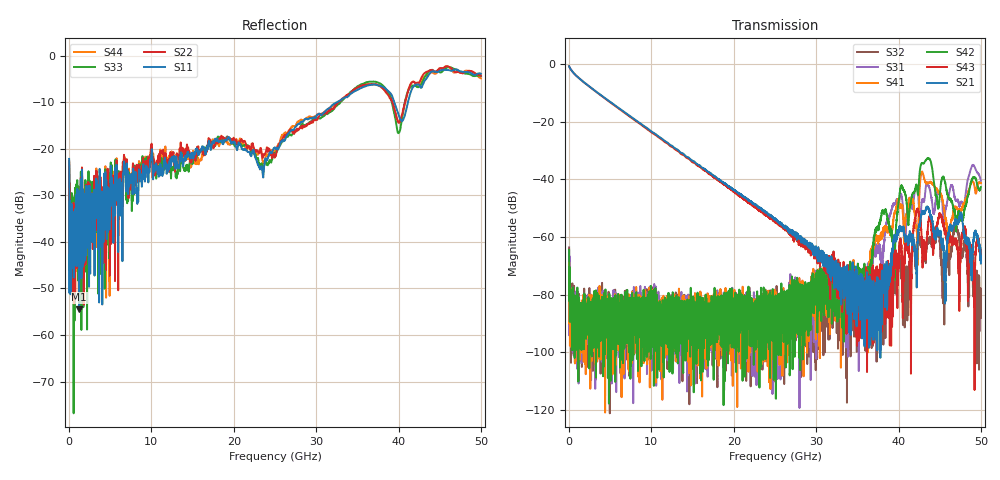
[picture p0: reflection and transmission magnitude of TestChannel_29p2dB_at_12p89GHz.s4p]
!Keysight Technologies,N5245A,MY49151038,A.10.64.09
!Date: Tuesday, July 23, 2019 14:25:50
!Correction: S11(Full 4 Port(1,2,3,4))
!S12(Full 4 Port(1,2,3,4))
!S13(Full 4 Port(1,2,3,4))
!S14(Full 4 Port(1,2,3,4))
!S21(Full 4 Port(1,2,3,4))
!S22(Full 4 Port(1,2,3,4))
!S23(Full 4 Port(1,2,3,4))
!S24(Full 4 Port(1,2,3,4))
!S31(Full 4 Port(1,2,3,4))
!S32(Full 4 Port(1,2,3,4))
!S33(Full 4 Port(1,2,3,4))
!S34(Full 4 Port(1,2,3,4))
!S41(Full 4 Port(1,2,3,4))
!S42(Full 4 Port(1,2,3,4))
!S43(Full 4 Port(1,2,3,4))
!S44(Full 4 Port(1,2,3,4))
!S4P File: Measurements: <S11,S12,S13,S14>,
!<S21,S22,S23,S24>,
!<S31,S32,S33,S34>,
!<S41,S42,S43,S44>:
# Hz S  MA  R 50
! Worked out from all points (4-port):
!   5000 points, 10 MHz to 50 GHz, reference 50 ohm
!   strongest paths, dB at 10 MHz, 12.51 GHz, 25.01 GHz, 37.51 GHz, 50 GHz:
!     S21: -0.7, -28.3, -54.0, -83.7, -69.2
!     S43: -0.6, -28.7, -54.8, -71.3, -67.5
!     S42: -64.5, -82.9, -85.5, -57.1, -42.6
!     S41: -69.0, -89.4, -89.9, -62.4, -41.1
!     S31: -64.8, -86.7, -84.3, -65.7, -40.4
!     S32: -63.6, -92.7, -90.6, -84.4, -78.2
!   lowest |S11| = -54.5 dB at 1.23 GHz (marker M1), VSWR 1.00, Z = 50.1 + j0.175 ohm
!   |S11| at or under -10 dB: start of sweep to 32.54 GHz; 39.5 GHz to 41.15 GHz (1.651 GHz wide, 4.09 % of centre)
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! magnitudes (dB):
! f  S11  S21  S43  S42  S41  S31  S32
! 10 MHz  -22.2  -0.7  -0.6  -64.5  -69.0  -64.8  -63.6
! 1.23 GHz  -54.5  -4.8  -4.9  -91.4  -81.8  -84.3  -104.1
! 34.74 GHz  -7.6  -79.4  -74.2  -72.8  -75.2  -80.5  -79.4
! 43.45 GHz  -4.8  -49.6  -61.1  -32.8  -41.4  -41.2  -62.5
! 46.08 GHz  -3.1  -59.0  -62.0  -46.4  -63.5  -45.3  -68.3
! 46.99 GHz  -3.0  -55.7  -61.7  -58.1  -49.5  -47.5  -57.6
! 50 GHz  -3.9  -69.2  -67.5  -42.6  -41.1  -40.4  -78.2
